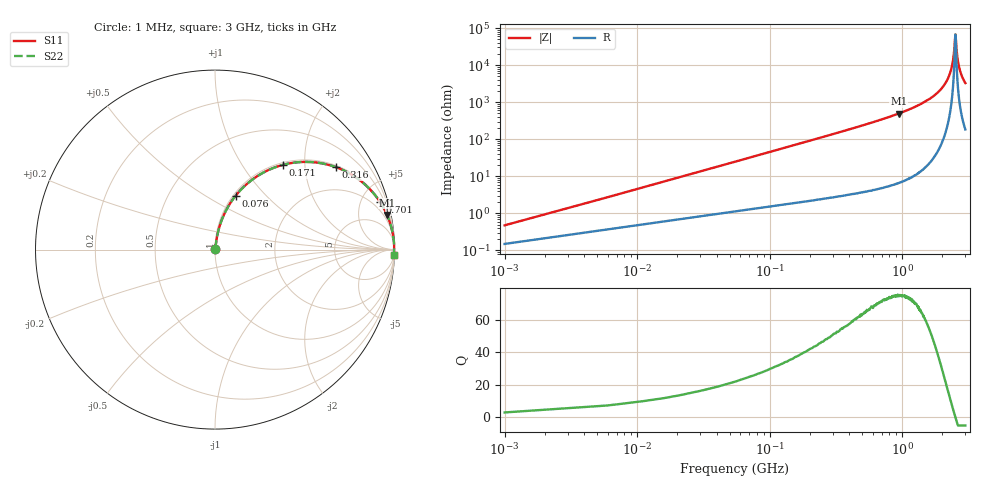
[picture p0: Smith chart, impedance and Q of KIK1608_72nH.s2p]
!version-2
!date-01.2022
!Series
# MHz S RI R 50
!Freq ReS11 ImS11 ReS21 ImS21 ReS12 ImS12 ReS22 ImS22
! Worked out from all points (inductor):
!   601 points, 1 MHz to 3 GHz, reference 50 ohm
!   read as one part in series: L = 72 nH near 16 MHz
!   highest Q = 75.2 at 941 MHz (marker M1), where L = 83.6 nH
!   self-resonance near 2.52 GHz
!   S11 on the Smith chart (normalised r, x): 1 MHz: 1.00, +0.01; 76 MHz: 1.03, +0.69; 171 MHz: 1.04, +1.55; 316 MHz: 1.06, +2.90; 701 MHz: 1.10, +6.87; 3 GHz: 5, -66
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1  0.00154 0.00451  0.9985 -0.00451  0.9985 -0.00451  0.00154 0.00451
21  0.0157 0.0929  0.9843 -0.0929  0.9843 -0.0929  0.0157 0.0929
26  0.021 0.1143  0.979 -0.1143  0.979 -0.1143  0.021 0.1143
46  0.0505 0.1956  0.9495 -0.1956  0.9495 -0.1956  0.0505 0.1956
76  0.1152 0.3005  0.8848 -0.3005  0.8848 -0.3005  0.1152 0.3005
171  0.3797 0.4726  0.6203 -0.4726  0.6203 -0.4726  0.3797 0.4726
316  0.6753 0.4587  0.3247 -0.4587  0.3247 -0.4587  0.6753 0.4587
501  0.8439 0.3552  0.1561 -0.3552  0.1561 -0.3552  0.8439 0.3552
701  0.9188 0.2662  0.0812 -0.2662  0.0812 -0.2662  0.9188 0.2662
941  0.9583 0.1933  0.0417 -0.1933  0.0417 -0.1933  0.9583 0.1933
1005  0.9648 0.1778  0.0352 -0.1778  0.0352 -0.1778  0.9648 0.1778
1505  0.9896 0.0934  0.0104 -0.0934  0.0104 -0.0934  0.9896 0.0934
2005  0.997 0.0404  0.00302 -0.0404  0.00302 -0.0404  0.997 0.0404
2210  0.9981 0.0232  0.00193 -0.0232  0.00193 -0.0232  0.9981 0.0232
2355  0.9984 0.012  0.00157 -0.012  0.00157 -0.012  0.9984 0.012
2445  0.9985 0.00546  0.00148 -0.00546  0.00148 -0.00546  0.9985 0.00546
2505  0.9985 0.00123  0.00147 -0.00123  0.00147 -0.00123  0.9985 0.00123
2530  0.9985 -0.000506  0.00147 0.000506  0.00147 0.000506  0.9985 -0.000506
2600  0.9985 -0.00527  0.00153 0.00527  0.00153 0.00527  0.9985 -0.00527
2695  0.9983 -0.0115  0.00168 0.0115  0.00168 0.0115  0.9983 -0.0115
2825  0.998 -0.0198  0.002 0.0198  0.002 0.0198  0.998 -0.0198
3000  0.9974 -0.0303  0.00263 0.0303  0.00263 0.0303  0.9974 -0.0303
